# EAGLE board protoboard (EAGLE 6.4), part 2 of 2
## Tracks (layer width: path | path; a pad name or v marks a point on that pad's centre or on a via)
A1
  Top 0.61: PIN1A.1 21.27,84.61 21.93,84.61 21.93,84.6 18.88,84.6
  Bottom 0.254: 21.25,75.25 21.25,75.37 21.21,75.37 21.21,75.27
  Bottom 0.406: 19,75.25 21.25,75.25 | 21.25,75.25 25.47,75.25 | 21.25,75.25 21.25,75.76 21.25,87.92 21.27,87.92
  Bottom 0.61: PIN1A.1 21.25,88.42 21.25,75.76 | 21.25,76.05 21.25,75.37
A2
  Top 0.305: 21.27,83.34 18.73,83.34
  Top 0.61: 21.91,83.34 18.73,83.34 17.46,83.34 17.46,88.42 PIN2A.1
  Bottom 0.254: 18,74.6 18,74.69
  Bottom 0.406: 25.53,74.6 18,74.6 18,74.82 18,88.41
  Bottom 0.61: PIN2A.1 18,88.42 18,74.82 | 18,74.98 18,74.69
A3
  Top 0.61: 21.91,82.07 16.51,82.07 16.51,90.96 PIN3A.1
  Bottom 0.254: 17.02,74.82 17.02,74.79
  Bottom 0.406: 25.47,73.95 17.02,73.95 17.02,74.79 | 18.73,90.98 PIN3A.1
  Bottom 0.61: 18.73,90.98 17.02,90.98 17.02,74.79 | 17.02,74.82 17.02,74.04
A4
  Top 0.61: 21.91,80.8 15.56,80.8 15.56,93.5 PIN4A.1
  Bottom 0.254: 16.05,73.91 16.04,73.91
  Bottom 0.406: 25.47,73.3 16.04,73.3 16.04,73.91 16.04,92.8
  Bottom 0.61: PIN4A.1 16.04,93.5 16.04,73.91 | 16.05,73.91 16.05,73.39
A5
  Top 0.61: 21.91,79.53 14.61,79.53 14.61,91.92 13.65,91.92 PIN5A.1
  Bottom 0.254: 15.07,73.55 15.07,73.52
  Bottom 0.406: 25.47,72.65 15.07,72.65 15.07,73.52 15.07,90.85
  Bottom 0.61: PIN5A.1 13.65,90.84 15.07,90.84 15.07,73.52 | 15.07,73.55 15.07,72.74
A6
  Top 0.61: 21.91,78.26 13.65,78.26 13.65,90.96 PIN6A.1
  Bottom 0.254: 14.1,72 14.1,72.09
  Bottom 0.406: 25.47,72 14.1,72 14.1,72.84
  Bottom 0.61: PIN6A.1 11.11,89.93 14.1,89.93 14.1,72.84 | 14.1,73.1 14.1,72.09
A7
  Top 0.61: 21.91,76.99 12.7,76.99 12.7,88.42 PIN7A.1
  Bottom 0.254: 13.12,71.35 13.12,71.44
  Bottom 0.406: 25.47,71.35 13.12,71.35 13.12,71.8 | PIN7A.1
  Bottom 0.61: PIN7A.1 13.12,88.41 13.12,71.8 | 13.12,71.93 13.12,71.44
A8
  Top 0.61: 21.91,75.72 11.75,75.72 11.75,85.88 PIN8A.1
  Bottom 0.254: 12.15,71.24 12.14,71.24 12.14,71.28
  Bottom 0.406: 25.47,70.7 12.14,70.7 12.14,71.18 | PIN8A.1
  Bottom 0.61: PIN8A.1 12.14,85.88 12.14,71.28 12.14,71.18 | 12.15,71.24 12.15,70.79
A9
  Top 0.61: 21.91,74.45 10.79,74.45 10.79,83.34 PIN9A.1
  Bottom 0.254: 11.17,70.14 11.17,70.17
  Bottom 0.406: 25.47,70.05 11.17,70.05 11.17,70.17 11.17,70.46 | PIN9A.1
  Bottom 0.61: PIN9A.1 11.17,83.34 11.17,70.46 | 11.17,70.66 11.17,70.14
A10
  Top 0.305: 20.64,73.18 19.68,73.18
  Top 0.61: PIN10A.1 9.84,80.8 9.84,73.18 19.68,73.18 21.91,73.18
  Bottom 0.254: 10.2,69.49 10.2,69.52
  Bottom 0.406: 25.47,69.4 10.2,69.4 10.2,69.52 10.2,69.85 10.2,80.81
  Bottom 0.61: PIN10A.1 10.2,80.8 10.2,69.85 | 10.2,69.98 10.2,69.49
A11
  Top 0.61: 21.91,71.91 8.89,71.91 8.89,78.26 PIN11A.1
  Bottom 0.254: 9.22,68.87 9.22,68.94
  Bottom 0.406: 25.47,68.75 9.22,68.75 9.22,68.94 9.22,69.62 9.22,78.27
  Bottom 0.61: PIN11A.1 9.22,78.26 9.22,69.62 | 9.22,69.94 9.22,68.87
A12
  Top 0.61: 21.91,70.64 7.94,70.64 7.94,75.72 PIN12A.1
  Bottom 0.254: 8.25,68.19 8.24,68.19 8.24,68.22
  Bottom 0.406: 25.47,68.1 8.24,68.1 8.24,68.22 8.24,68.87 8.24,75.7
  Bottom 0.61: PIN12A.1 8.24,75.72 8.24,68.87 | 8.25,69 8.25,68.19
A13
  Top 0.305: 6.98,73.18 6.67,73.18
  Top 0.61: 21.91,69.37 6.98,69.37 6.98,73.18 | 6.67,73.18 PIN13A.1 6.07,73.18 6.07,73.17
  Bottom 0.406: 25.47,67.45 7.27,67.45 7.27,67.67 7.27,68.12
  Bottom 0.61: 6.03,73.17 6.1,73.17 | 6.1,73.17 7.27,73.17 7.27,68.12 | 7.27,68.29 7.27,67.67 | 7.27,67.57 7.27,67.67 | 7.27,67.67 | PIN13A.1 6.1,73.18 6.1,73.17
A14
  Top 0.61: 21.91,68.1 6.03,68.1 6.03,70.64 PIN14A.1
  Bottom 0.254: 6.3,66.89 6.29,66.89 6.29,66.95
  Bottom 0.406: 25.47,66.8 6.29,66.8 6.29,66.95 6.29,67.28 6.29,70.63
  Bottom 0.61: PIN14A.1 6.29,70.64 6.29,67.28 | 6.3,67.47 6.3,66.89
A15
  Top 0.61: 21.91,66.83 5.08,66.83 5.08,68.1 PIN15A.1
  Bottom 0.254: 5.32,66.24 5.32,66.27
  Bottom 0.406: 25.47,66.15 5.32,66.15 5.32,66.27 5.32,66.73
  Bottom 0.61: 5.32,66.73 5.32,68.1 PIN15A.1 | 5.32,66.86 5.32,66.24
A16
  Top 0.61: 21.91,65.56 PIN16A.1
  Bottom 0.406: 25.47,65.5 4.9,65.5 4.34,65.5
  Bottom 0.61: PIN16A.1 3.49,65.5 4.9,65.5
A17
  Top 0.61: 21.91,64.29 5.08,64.29 5.08,63.02 PIN17A.1
  Bottom 0.406: 25.47,64.85 5.32,64.85 5.32,64.75
  Bottom 0.61: 5.32,64.75 5.32,63.02 PIN17A.1
A18
  Top 0.61: 21.91,63.02 6.03,63.02 6.03,60.48 PIN18A.1
  Bottom 0.254: 6.3,64.09 6.29,64.09
  Bottom 0.406: 25.47,64.2 6.29,64.2 6.29,64.09 6.29,63.67 6.29,60.62
  Bottom 0.61: PIN18A.1 6.29,60.48 6.29,63.67 | 6.3,63.54 6.3,64.09
A19
  Top 0.61: 21.91,61.75 6.98,61.75 6.98,57.94 PIN19A.1
  Bottom 0.254: 7.27,62.99 7.27,63.02
  Bottom 0.406: 25.47,63.55 7.27,63.55 7.27,63.05 | 7.27,63.02 7.27,58.25
  Bottom 0.61: PIN19A.1 7.27,57.94 7.27,63.02 7.27,63.05 | 7.27,62.99 7.27,63.44
A20
  Top 0.61: 21.91,60.48 7.94,60.48 7.94,55.4 PIN20A.1
  Bottom 0.254: 8.25,62.79 8.24,62.79 8.24,62.76
  Bottom 0.305: 6.03,55.42 PIN20A.1
  Bottom 0.406: 25.47,62.9 8.24,62.9 8.24,62.76 8.24,62.37
  Bottom 0.61: 6.03,55.42 8.24,55.42 8.24,62.37 | 8.25,62.08 8.25,62.79
A21
  Top 0.61: 21.91,59.21 8.89,59.21 8.89,52.86 PIN21A.1
  Bottom 0.254: 9.22,62.25 9.22,62.14
  Bottom 0.406: 25.47,62.25 9.22,62.25 9.22,61.75 9.22,52.82
  Bottom 0.61: PIN21A.1 9.22,52.86 9.22,61.75 | 9.22,61.62 9.22,62.14
A22
  Top 0.61: 21.91,57.94 9.84,57.94 9.84,50.32 PIN22A.1
  Bottom 0.254: 10.2,61.49 10.29,61.49 10.29,61.6
  Bottom 0.406: 25.47,61.6 10.29,61.6 10.2,61.6 10.2,61.1 10.2,50.45
  Bottom 0.61: PIN22A.1 10.2,50.32 10.2,61.1 | 10.2,60.88 10.2,61.49
A23
  Top 0.61: 21.91,56.67 10.79,56.67 10.79,47.78 PIN23A.1
  Bottom 0.254: 11.17,60.45 11.17,60.49
  Bottom 0.406: 25.47,60.95 11.17,60.95 11.17,60.49 11.17,60.42 11.17,47.95
  Bottom 0.61: PIN23A.1 11.17,47.78 11.17,60.42 | 11.17,60.45 11.17,60.84
A24
  Top 0.61: 21.91,55.4 11.75,55.4 11.75,45.24 9.21,45.24 PIN24A.1
  Bottom 0.254: 12.14,59.8 12.15,59.8 12.15,59.77
  Bottom 0.406: 25.47,60.3 12.14,60.3 12.14,59.8
  Bottom 0.61: PIN24A.1 12.14,45.24 12.14,59.8 | 12.15,59.71 12.15,59.77 12.15,60.19
A25
  Top 0.61: 21.91,54.13 12.7,54.13 12.7,42.7 PIN25A.1
  Bottom 0.254: 13.12,59.06 13.12,59.02
  Bottom 0.406: 25.47,59.65 13.12,59.65 13.12,59.06 13.12,42.75
  Bottom 0.61: PIN25A.1 13.12,42.7 13.12,59.06 | 13.12,59.02 13.12,59.54
A26
  Top 0.61: 21.91,52.86 13.65,52.86 13.65,40.16 PIN26A.1
  Bottom 0.254: 14.1,58.5 14.1,58.57
  Bottom 0.406: 25.47,59 14.1,59 14.1,58.5
  Bottom 0.61: PIN26A.1 11.11,41.45 14.1,41.45 14.1,58.5 | 14.1,58.57 14.1,58.89
A27
  Top 0.61: 21.84,51.59 14.61,51.59 14.61,39.21 13.65,39.21 PIN27A.1
  Bottom 0.254: 15.07,57.92 15.07,57.98
  Bottom 0.406: 25.47,58.35 15.07,58.35 15.07,57.98 15.07,40.47
  Bottom 0.61: PIN27A.1 13.65,40.47 15.07,40.47 15.07,57.98 | 15.07,57.92 15.07,58.24
A28
  Top 0.61: 21.84,50.32 15.56,50.32 15.56,37.62 PIN28A.1
  Bottom 0.254: 16.05,57.11 16.04,57.11 16.04,57.17
  Bottom 0.406: 25.47,57.7 16.04,57.7 16.04,57.17 16.04,38.52
  Bottom 0.61: PIN28A.1 16.04,37.62 16.04,57.17 | 16.05,57.11 16.05,57.59
A29
  Top 0.61: 21.84,49.05 16.51,49.05 16.51,40.16 PIN29A.1
  Bottom 0.254: 17.02,56.94
  Bottom 0.305: 17.05,57.04 17.02,57.04 17.02,56.99
  Bottom 0.406: 17.02,57.05 17.02,56.99 17.02,56.94 17.02,56.49 17.02,40.15 | 17.05,57.04 25.44,57.04
  Bottom 0.61: PIN29A.1 17.02,40.16 17.02,56.49 | 17.02,56.42 17.02,56.94
A30
  Top 0.61: 21.84,47.78 17.46,47.78 17.46,42.7 PIN30A.1
  Bottom 0.254: 18,55.87
  Bottom 0.305: 18,56.4 18.03,56.4 18.03,56.39
  Bottom 0.406: 18,56.4 18,55.87 18,42.75 | 18.03,56.39 25.44,56.39
  Bottom 0.61: PIN30A.1 18,42.7 18,55.87 | 18,55.87 18,56.29
A31
  Top 0.61: 18.67,46.51 21.27,46.51 | 21.27,46.51 21.91,46.51 | PIN31A.1 21.27,46.51
  Bottom 0.254: 21.21,55.74 21.25,55.74 21.25,55.58
  Bottom 0.305: 21.25,55.75 21.27,55.75 21.27,55.74
  Bottom 0.406: 18.97,55.75 21.25,55.75 21.25,55.25 21.25,43.72 | 21.21,55.74 21.27,55.74 25.44,55.74
  Bottom 0.61: PIN31A.1 21.25,42.7 21.25,55.25 | 21.25,54.99 21.25,55.58
B1
  Top 0.61: 33.97,84.61 31.43,84.61 | 31.43,84.61 23.18,84.61 | 31.43,84.61 PIN1B.1
  Bottom 0.254: 31.64,76.15 31.65,76.15
  Bottom 0.406: 27.42,75.25 31.64,75.25 | 31.64,75.25 34.19,75.25 | 31.64,87.6 31.64,76.15 31.64,75.25
  Bottom 0.61: PIN1B.1 31.64,88.42 31.64,76.15 | 31.65,76.15 31.65,75.44
B2
  Top 0.61: 23.18,83.34 35.24,83.34 35.24,88.42 PIN2B.1
  Bottom 0.254: 34.9,76.15 34.9,76.12
  Bottom 0.406: 27.42,74.6 34.9,74.6 34.9,76.15 34.9,88.25
  Bottom 0.61: PIN2B.1 34.9,88.42 34.9,76.15 | 34.9,76.51 34.9,76.12 34.9,75.7
B3
  Top 0.61: PIN3B.1 36.2,90.96 36.2,82.07 23.18,82.07
  Bottom 0.254: 35.87,74.75
  Bottom 0.406: 27.42,73.95 35.87,73.95 35.87,74.75 35.87,90.85
  Bottom 0.61: PIN3B.1 35.87,90.96 35.87,74.75 | 35.87,74.82 35.87,74.75 35.87,74.04
B4
  Top 0.61: 23.18,80.8 37.15,80.8 37.15,93.5 PIN4B.1
  Bottom 0.254: 36.85,74.07 36.85,74.01
  Bottom 0.406: 27.42,73.3 36.85,73.3 36.85,74.07 36.85,92.8
  Bottom 0.61: PIN4B.1 36.85,93.5 36.85,74.07 | 36.85,74.1 36.85,74.01 36.85,73.39
B5
  Top 0.61: 23.18,79.53 38.1,79.53 38.1,91.92 39.05,91.92 PIN5B.1
  Bottom 0.406: 27.42,72.65 37.82,72.65 37.82,73.62 37.82,90.85
  Bottom 0.61: PIN5B.1 39.05,91.49 37.82,91.49 37.82,73.62 | 37.82,73.62 | 37.82,73.62 37.82,72.74
B6
  Top 0.61: PIN6B.1 39.05,90.96 39.05,78.26 23.18,78.26
  Bottom 0.254: 38.8,72.41 38.8,72.45
  Bottom 0.406: 27.42,72 38.8,72 38.8,72.41 38.8,89.55
  Bottom 0.61: PIN6B.1 41.59,89.54 38.8,89.54 38.8,72.41 | 38.8,72.45 38.8,72.09
B7
  Top 0.61: PIN7B.1 40.01,88.42 40.01,76.99 23.18,76.99
  Bottom 0.254: 39.77,71.35 39.77,71.44
  Bottom 0.406: 27.42,71.35 39.77,71.35 39.77,72.28 39.77,88.25
  Bottom 0.61: PIN7B.1 39.77,88.42 39.77,72.28 | 39.77,73.36 39.77,71.44
B8
  Top 0.61: 23.18,75.72 40.96,75.72 40.96,85.88 PIN8B.1
  Bottom 0.406: 27.42,70.7 40.75,70.7 40.75,70.79 40.75,85.97
  Bottom 0.61: PIN8B.1 40.75,85.88 40.75,70.79
B9
  Top 0.61: 23.18,74.45 41.91,74.45 41.91,83.34 PIN9B.1
  Bottom 0.254: 41.72,70.05 41.72,70.14
  Bottom 0.406: 27.42,70.05 41.72,70.05 41.72,70.82 | PIN9B.1 44.13,83.37
  Bottom 0.61: 44.13,83.37 41.72,83.37 41.72,70.82 | 41.72,70.95 41.72,70.14
B10
  Top 0.61: 23.18,73.18 42.86,73.18 42.86,80.8 PIN10B.1
  Bottom 0.254: 42.7,69.49 42.7,69.46
  Bottom 0.406: 27.42,69.4 42.7,69.4 42.7,69.46 42.7,69.85 | 44.13,80.77 PIN10B.1
  Bottom 0.61: 44.13,80.77 42.7,80.77 42.7,69.85 | 42.7,69.98 42.7,69.49
B11
  Top 0.61: 23.18,71.91 43.82,71.91 43.82,78.26 PIN11B.1
  Bottom 0.305: 46.67,78.17 PIN11B.1
  Bottom 0.406: 27.42,68.75 43.67,68.75 43.67,78.17
  Bottom 0.61: 43.67,78.17 45.95,78.17 46.67,78.17
B12
  Top 0.61: 23.18,70.64 44.77,70.64 44.77,75.72 PIN12B.1
  Bottom 0.254: 44.65,68.19
  Bottom 0.406: 27.42,68.1 44.65,68.1 44.65,68.19 44.65,68.58 44.65,75.57
  Bottom 0.61: PIN12B.1 44.65,75.72 44.65,68.58 | 44.65,68.81 44.65,68.19
B13
  Top 0.61: 23.18,69.37 45.72,69.37 45.72,73.18 PIN13B.1
  Bottom 0.254: 45.62,68.09
  Bottom 0.406: 27.42,67.45 45.62,67.45 45.62,68.03 | 45.62,68.09 45.62,72.65
  Bottom 0.61: PIN13B.1 45.62,73.18 45.62,68.09 45.62,68.03 | 45.62,68.09 45.62,67.54
B14
  Top 0.61: 23.18,68.1 46.67,68.1 46.67,70.64 PIN14B.1
  Bottom 0.254: 46.6,66.89
  Bottom 0.406: 27.42,66.8 46.6,66.8 46.6,66.89 46.6,67.31 46.6,70.7
  Bottom 0.61: PIN14B.1 46.6,70.64 46.6,67.31 | 46.6,67.54 46.6,66.89
B15
  Top 0.61: 23.18,66.83 47.62,66.83 47.62,68.1 PIN15B.1
  Bottom 0.254: 47.57,66.73 47.57,66.69
  Bottom 0.406: 27.42,66.15 47.57,66.15 47.57,66.63 | PIN15B.1
  Bottom 0.61: PIN15B.1 47.57,68.1 47.57,66.69 47.57,66.63 | 47.57,66.73 47.57,66.24
B16
  Top 0.61: 23.18,65.56 PIN16B.1
  Bottom 0.406: 27.42,65.5 48,65.5 48.55,65.5 | 49.21,65.5 PIN16B.1
  Bottom 0.61: 49.21,65.5 48,65.5
B17
  Top 0.61: 23.18,64.29 47.62,64.29 47.62,63.02 PIN17B.1
  Bottom 0.254: 47.57,64.29 47.57,64.26
  Bottom 0.406: 27.42,64.85 47.57,64.85 47.57,64.65 | 47.57,64.26 47.57,63.09
  Bottom 0.61: PIN17B.1 47.57,63.02 47.57,64.26 47.57,64.65 | 47.57,64.29 47.57,64.74
B18
  Top 0.61: 23.18,63.02 46.67,63.02 46.67,60.48 PIN18B.1
  Bottom 0.254: 46.6,64.2 46.6,64.09
  Bottom 0.406: 27.42,64.2 46.6,64.2 46.6,63.31 46.6,60.82
  Bottom 0.61: PIN18B.1 46.6,60.48 46.6,63.31 | 46.6,62.89 46.6,64.09
B19
  Top 0.61: 23.18,61.75 45.72,61.75 45.72,57.94 PIN19B.1
  Bottom 0.254: 45.62,62.96 45.62,62.99
  Bottom 0.406: 27.42,63.55 45.62,63.55 45.62,62.96 45.62,58.35
  Bottom 0.61: PIN19B.1 45.62,57.94 45.62,62.96 | 45.62,62.89 45.62,62.99 45.62,63.44
B20
  Top 0.61: 23.18,60.48 44.77,60.48 44.77,55.4 PIN20B.1
  Bottom 0.254: 44.65,62.9 44.65,62.79
  Bottom 0.406: 27.42,62.9 44.65,62.9 44.65,62.44 44.65,55.42
  Bottom 0.61: PIN20B.1 44.65,55.4 44.65,62.44 | 44.65,62.24 44.65,62.79
B21
  Top 0.61: PIN21B.1 43.82,52.86 43.82,59.21 23.18,59.21
  Bottom 0.254: 43.67,62.25 43.67,62.14
  Bottom 0.406: 27.42,62.25 43.67,62.25 43.67,61.75 43.67,53.31 | 46.67,52.82 PIN21B.1
  Bottom 0.61: 46.67,52.82 43.67,52.82 43.67,61.75 | 43.67,61.53 43.67,62.14
B22
  Top 0.61: 23.18,57.94 42.86,57.94 42.86,50.32 PIN22B.1
  Bottom 0.254: 42.7,61.6 42.7,61.49
  Bottom 0.406: 27.42,61.6 42.7,61.6 42.7,60.75 42.7,50.55
  Bottom 0.61: PIN22B.1 42.7,50.32 42.7,60.75 | 42.7,60.26 42.7,61.49
B23
  Top 0.61: PIN23B.1 41.91,47.78 41.91,56.67 23.18,56.67
  Bottom 0.254: 41.72,60.84 41.72,60.88
  Bottom 0.406: 27.42,60.95 41.72,60.95 41.72,60.88 41.72,60.52 41.72,47.95
  Bottom 0.61: PIN23B.1 41.72,47.78 41.72,60.52 | 41.72,60.19 41.72,60.84
B24
  Top 0.61: 23.18,55.4 40.96,55.4 40.96,45.24 PIN24B.1
  Bottom 0.254: 40.75,60.3 40.75,60.19
  Bottom 0.406: 27.42,60.3 40.75,60.3 40.75,59.8 40.75,45.35
  Bottom 0.61: PIN24B.1 40.75,45.24 40.75,59.8 | 40.75,59.48 40.75,60.19
B25
  Top 0.61: PIN25B.1 40.01,42.7 40.01,54.13 23.18,54.13
  Bottom 0.254: 39.77,59.65 39.77,59.54
  Bottom 0.406: 27.42,59.65 39.77,59.65 39.77,59.15 39.77,43.07
  Bottom 0.61: PIN25B.1 39.77,42.7 39.77,59.15 | 39.77,58.86 39.77,59.54
B26
  Top 0.61: 23.18,52.86 39.05,52.86 39.05,40.16 PIN26B.1
  Bottom 0.254: 38.8,59 38.8,58.89
  Bottom 0.406: 27.42,59 38.8,59 38.8,58.54 38.8,41.45
  Bottom 0.61: PIN26B.1 41.59,41.44 38.8,41.44 38.8,58.54 | 38.8,58.34 38.8,58.89
B27
  Top 0.61: 23.18,51.59 38.1,51.59 38.1,38.89 39.05,38.89 PIN27B.1
  Bottom 0.254: 37.82,58.35 37.82,58.24
  Bottom 0.406: 27.42,58.35 37.82,58.35 37.82,57.85 37.82,40.15
  Bottom 0.61: PIN27B.1 39.05,40.14 37.82,40.14 37.82,57.85 | 37.82,57.72 37.82,58.24
B28
  Top 0.61: 23.18,50.32 37.15,50.32 37.15,37.62 PIN28B.1
  Bottom 0.254: 36.85,57.59 36.85,57.63
  Bottom 0.406: 27.42,57.7 36.85,57.7 36.85,57.63 36.85,57.37 36.85,38.2
  Bottom 0.61: PIN28B.1 36.85,37.62 36.85,57.37 | 36.85,57.24 36.85,57.59
B29
  Top 0.61: 23.18,49.05 36.2,49.05 36.2,40.16 PIN29B.1 34.02,40.16 34.02,40.15 | 34.02,40.15 33.97,40.15 | 35.03,40.15 34.54,40.15 34.02,40.15
  Bottom 0.254: 33.97,40.15 PIN29B.1
  Bottom 0.406: 34.57,40.15 35.87,40.15 35.87,57.05 35.88,57.05 35.88,56.36 35.91,56.36 35.91,56.42 | 27.45,57.04 35.91,57.04 35.91,56.94
  Bottom 0.61: 33.97,40.15 35.91,40.15 35.91,56.42 35.91,56.94
B30
  Top 0.61: 23.18,47.78 35.24,47.78 35.24,42.7 PIN30B.1
  Bottom 0.254: 34.9,56.39 34.9,56.4
  Bottom 0.406: 34.9,56.39 27.45,56.39 | 34.9,56.4 34.9,55.29 34.9,43.07
  Bottom 0.61: PIN30B.1 34.9,42.7 34.9,55.29
B31
  Top 0.61: PIN31B.1 31.43,46.51 | 31.43,46.51 33.97,46.51 | 23.18,46.51 31.43,46.51
  Bottom 0.254: 31.65,55.58 31.65,55.74 31.65,55.75
  Bottom 0.406: 34.12,55.75 31.65,55.75 31.64,55.75 31.64,55.42 31.64,43.4 | 31.75,55.74 31.65,55.74 27.45,55.74
  Bottom 0.61: PIN31B.1 31.64,42.7 31.64,55.42 | 31.65,54.8 31.65,55.58
BOK1  (via drill 0.7)
  Top 2.184: 11.11,93.82 v11.11,97.31
  Bottom 0.406: PIN-BOK1.1 11.17,93.5 11.17,93.28 11.11,93.28 11.11,93.82
  Bottom 2.184: v11.11,97.31 11.11,93.82
BOK2  (via drill 0.7)
  Top 2.184: 18.73,93.82 v18.73,97.31
  Bottom 0.406: PIN-BOK2.1 18.73,93.82
  Bottom 2.184: v18.73,97.31 18.73,93.82
BOK3  (via drill 0.7)
  Top 2.184: 21.27,93.82 v21.27,97.31
  Bottom 0.406: PIN-BOK3.1 21.27,93.82
  Bottom 2.184: v21.27,97.31 21.27,93.82
BOK4  (via drill 0.7)
  Top 2.184: 23.81,93.82 v23.81,97.31
  Bottom 0.406: PIN-BOK4.1 23.81,93.82
  Bottom 2.184: v23.81,97.31 23.81,93.82
BOK5  (via drill 0.7)
  Top 2.184: 26.35,93.82 v26.35,97.31
  Bottom 0.406: PIN-BOK5.1 26.35,93.82
  Bottom 2.184: v26.35,97.31 26.35,93.82
BOK6  (via drill 0.7)
  Top 2.184: 28.89,93.82 v28.89,97.31
  Bottom 0.61: 28.89,96.04 PIN-BOK6.1 v28.89,97.31
  Bottom 2.184: v28.89,97.31 28.89,96.04 28.89,93.82
BOK7  (via drill 0.7)
  Top 2.184: 31.43,93.82 v31.43,97.31
  Bottom 2.184: v31.43,97.31 PIN-BOK7.1
BOK8  (via drill 0.7)
  Top 2.184: PIN-BOK8.1 v33.97,97.31
  Bottom 2.184: v33.97,97.31 33.97,93.82
BOK9  (via drill 0.7)
  Top 2.184: PIN-BOK9.1 v41.59,97.31
  Bottom 2.184: v41.59,97.31 41.59,93.82
BOK10  (via drill 0.7)
  Top 2.184: PIN-BOK10.1 v44.13,97.31
  Bottom 2.184: v44.13,97.31 44.13,93.82
BOK11  (via drill 0.7)
  Top 2.184: PIN-BOK11.1 v46.67,97.31
  Bottom 2.184: v46.67,97.31 46.67,93.82
BOK12  (via drill 0.7)
  Top 2.184: PIN-BOK12.1 v49.21,97.31
  Bottom 2.184: v49.21,97.31 49.21,93.82
C1
  Top 0.61: IC2.4 18.73,30.95 18.73,32.44 16.19,32.44 PIN1C.1
  Bottom 0.305: 22.32,32.44 22.32,30.84 22.32,23.34 22.54,23.34 | 22.32,23.34 22.54,23.34 | 22.54,23.34 31.96,23.34
  Bottom 0.61: PIN1C.1 22.32,32.54 22.32,30.84
C2
  Top 0.61: IC2.5 PIN2C.1
  Bottom 0.305: 21.91,22.83 21.59,22.83 | 21.59,22.83 21.53,22.83 21.53,28.34 | 31.96,22.84 21.59,22.84 21.59,22.83
  Bottom 0.61: PIN2C.1 21.53,30 21.53,28.34
C3
  Top 0.61: IC2.6 18.73,29.05 18.73,27.56 16.19,27.56 PIN3C.1
  Bottom 0.254: PIN3C.1
  Bottom 0.305: 20.82,25.84 20.82,22.34 31.96,22.34
  Bottom 0.61: PIN3C.1 20.82,27.47 20.82,25.84
C4
  Top 0.813: PIN4C.1 29.53,24.92 U6.P_POUZDRO
  Bottom 0.254: PIN4C.1 16.96,24.92 16.96,24.94
  Bottom 0.305: 20.07,23.84 20.07,21.84 20.32,21.84 | 20.07,21.84 20.32,21.84 | 20.32,21.84 31.96,21.84
  Bottom 0.61: 16.19,24.94 16.96,24.94 20.07,24.94 20.07,23.84
C5
  Top 0.813: PIN5C.1 23.33,22.38 U6.P_A
  Bottom 0.305: 19.32,22.38 19.32,21.84 19.32,21.34 31.96,21.34
  Bottom 0.61: PIN5C.1 19.32,22.38 19.32,21.84
C6
  Top 0.813: U6.P-B PIN6C.1
  Bottom 0.254: PIN6C.1 16.46,19.84 16.46,19.81
  Bottom 0.305: 19.32,20.34 19.32,20.84 31.96,20.84
  Bottom 0.61: 16.19,19.81 16.46,19.81 19.32,19.81 19.32,20.34
C7
  Top 0.813: PIN7C.1 23.33,17.3 U6.P-C
  Bottom 0.254: PIN7C.1 16.46,17.3 16.46,17.31
  Bottom 0.305: 20.07,20.34 20.07,18.84 | 20.07,20.35 20.07,20.34 | 20.07,20.34 31.96,20.34
  Bottom 0.61: 16.19,17.31 16.46,17.31 20.07,17.31 20.07,18.84
C8
  Top 0.61: U1.1 18.41,13.8 18.41,14.69 16.19,14.69 PIN8C.1
  Bottom 0.254: PIN8C.1
  Bottom 0.305: 20.82,15.84 20.82,19.84 31.96,19.84
  Bottom 0.61: PIN8C.1 20.82,14.75 20.82,15.84
C9
  Top 0.61: U1.2 PIN9C.1
  Bottom 0.254: 16.19,12.19 PIN9C.1
  Bottom 0.305: 21.57,13.84 21.57,19.34 31.96,19.34
  Bottom 0.61: 16.19,12.19 21.57,12.19 21.57,13.84
C10
  Top 0.61: U1.3 18.41,10.52 18.41,9.56 16.16,9.56 PIN10C.1
  Bottom 0.305: 22.32,9.66 22.32,11.34 22.32,18.83 31.96,18.83 31.96,18.84
  Bottom 0.61: PIN10C.1 22.32,9.65 22.32,11.34
D1
  Top 0.406: IC1.3 46.04,30.65 46.04,31.59 | 49.21,32.6 PIN1D.1
  Top 0.61: 46.04,31.59 46.04,32.6 49.21,32.6
  Bottom 0.254: PIN1D.1
  Bottom 0.305: 43.82,31.34 43.82,23.34 32.78,23.34
  Bottom 0.61: PIN1D.1 43.82,32.53 43.82,31.34
D2
  Top 0.406: IC1.2 46.67,30
  Top 0.61: PIN2D.1 46.67,30
  Bottom 0.254: PIN2D.1
  Bottom 0.305: 44.57,29.34 44.57,22.84 32.78,22.84
  Bottom 0.61: PIN2D.1 44.57,30 44.57,29.34
D3
  Top 0.406: IC1.1 46.04,29.35 46.04,28.26
  Top 0.61: 46.04,28.26 46.04,27.46 PIN3D.1
  Bottom 0.305: 45.28,26.84 45.28,22.34 32.78,22.34
  Bottom 0.61: PIN3D.1 45.28,27.46 45.28,26.84
D4
  Top 0.813: U7.P_POUZDRO 34.72,24.92 PIN4D.1
  Bottom 0.305: 46.07,24.91 46.07,23.84 46.07,21.84 32.78,21.84
  Bottom 0.61: PIN4D.1 46.07,24.92 46.07,23.84
D5
  Top 0.813: U7.P-A 42.02,22.38 PIN5D.1
  Bottom 0.305: 46.82,22.38 46.82,21.84 46.82,21.34 32.78,21.34
  Bottom 0.61: PIN5D.1 46.82,22.38 46.82,21.84
D6
  Top 0.813: U7.P-B PIN6D.1
  Bottom 0.254: PIN6D.1 48.97,19.84
  Bottom 0.305: 46.82,20.34 46.82,20.81 46.67,20.81 46.67,20.84 | 46.82,20.84 46.67,20.84 | 46.67,20.84 32.78,20.84
  Bottom 0.61: PIN6D.1 48.97,19.84 46.82,19.84 46.82,20.34
D7
  Top 0.813: U7.P-C 42.02,17.3 PIN7D.1
  Bottom 0.305: 46.07,17.31 46.07,18.84 46.07,20.34 32.78,20.34
  Bottom 0.61: PIN7D.1 46.07,17.3 46.07,18.84
D8
  Top 0.61: U2.6 46.04,13.92 46.04,14.81 49.21,14.81 PIN8D.1
  Bottom 0.254: PIN8D.1 48.97,14.76 48.97,14.75
  Bottom 0.305: 45.32,15.84 45.32,19.81 45.09,19.81 45.09,19.84 | 32.78,19.84 45.09,19.84 | 45.09,19.84 45.32,19.84
  Bottom 0.61: PIN8D.1 48.97,14.75 45.32,14.75 45.32,15.84
D9
  Top 0.61: U2.5 PIN9D.1
  Bottom 0.254: PIN9D.1 48.97,12.22
  Bottom 0.305: 44.57,13.34 44.57,19.31 44.45,19.31 44.45,19.34 | 44.57,19.34 44.45,19.34 | 44.45,19.34 32.78,19.34
  Bottom 0.61: PIN9D.1 48.97,12.22 44.57,12.22 44.57,13.34
D10
  Top 0.61: U2.4 46.36,10.52 46.36,9.69 PIN10D.1
  Bottom 0.305: 43.82,9.69 43.82,10.84 43.82,18.84 32.78,18.84
  Bottom 0.61: PIN10D.1 43.82,9.68 43.82,10.84
IO/A
  Bottom 1.27: ARK-A.1 K1.1
IO/B
  Bottom 1.27: ARK-B.1 K1.2
IO/C
  Top 0.813: J-LED1A.1 84.77,96.52 K1.3
  Bottom 1.27: ARK-C.1 K1.3
IO/D
  Top 0.813: J-LED2A.1 66.99,93.98 66.99,95.41 79.69,95.41 K2.1
  Bottom 1.27: ARK-D.1 K2.1
IO/E
  Top 0.813: ARK-E.1 74.61,89.38 66.99,89.38 66.99,91.44 J-LED3A.1
  Bottom 1.27: ARK-E.1 K2.2
IO/F
  Top 0.813: ARK-F.1 65.09,86.04 J-LED4A.1
  Bottom 1.27: ARK-F.1 K2.3
J-2MM-A1  (via drill 0.9 pad 1.68)
  other vias: 8.2,38.32
J-2MM-A2  (via drill 0.9 pad 1.68)
  other vias: 8.2,36.32
J-2MM-A3  (via drill 0.9 pad 1.68)
  other vias: 8.2,34.32
J-2MM-A4  (via drill 0.9 pad 1.68)
  other vias: 8.2,32.33
J-2MM-B1  (via drill 0.9 pad 1.68)
  other vias: 3.2,38.32
J-2MM-B2  (via drill 0.9 pad 1.68)
  other vias: 3.2,36.32
J-2MM-B3  (via drill 0.9 pad 1.68)
  other vias: 3.19,34.33
J-2MM-B4  (via drill 0.9 pad 1.68)
  other vias: 3.2,32.32
LED1A
  Top 1.27: LED1.A J-LED1B.1
  Top 1.422: 59.37,96.52 LED1.A
LED2A
  Top 1.27: LED2.A J-LED2B.1
  Top 1.422: LED2.A 59.37,93.98
LED3A
  Top 1.27: LED3.A J-LED3B.1
  Top 1.422: LED3.A 59.37,91.44
LED4A
  Top 1.27: LED4.A J-LED4B.1
  Top 1.422: LED4.A 59.37,88.9
LEDK1
  Top 1.27: RLED1.2 LED1.C
LEDK2
  Top 1.27: RLED2.2 LED2.C
LEDK3
  Top 1.27: RLED3.2 LED3.C
LEDK4
  Top 1.27: RLED4.2 LED4.C
LEDNAP-K
  Top 1.27: LED-NAP.C RLED-NAP.2
POT1
  Bottom 0.813: PINPOT1B.1 PINPOT1A.1
POT2
  Bottom 0.813: PINPOT2B.1 PINPOT2A.1
SOT1
  Top 0.61: IC2.3 24.13,30.95 24.13,32.54 PIN-SOT1.1
SOT2
  Top 0.406: 23.81,30 24.66,30 25.4,30
  Top 0.61: IC2.2 24.66,30 PIN-SOT2.1
SOT3
  Top 0.406: 24.45,27.46 25.4,27.46
  Top 0.61: IC2.1 23.81,29.05 23.81,27.46 24.45,27.46 PIN-SOT3.1
SOT4
  Top 0.61: U1.6 26.67,13.92 26.67,14.76 PIN-SOT4.1
SOT5
  Top 0.61: U1.5 PIN-SOT5.1
SOT6
  Top 0.61: U1.4 26.67,10.52 26.67,9.68 PIN-SOT6.1
SOT7
  Top 0.406: IC1.4 41.59,30.65 41.59,31.75
  Top 0.61: PIN-SOT7.1 41.59,32.54 41.59,31.75
SOT8
  Top 0.406: 40.8,30 40.8,29.99 | 39.05,29.99 PIN-SOT8.1 | IC1.5 40.32,29.99
  Top 0.61: 40.8,29.99 40.32,29.99 39.05,29.99
SOT9
  Top 0.406: IC1.6 41.59,29.35 41.59,28.26
  Top 0.61: PIN-SOT9.1 41.59,27.46 41.59,28.26
SOT10
  Top 0.61: U2.1 38.42,13.8 38.42,14.76 PIN-SOT10.1
SOT11
  Top 0.61: U2.2 PIN-SOT11.1
SOT12
  Top 0.61: U2.3 38.42,10.52 38.42,9.68 PIN-SOT12.1
TINY-B0
  Bottom 1.27: JP24.1 J-B4.1
TINY-B1
  Bottom 1.27: JP21.1 J-B5.1
TINY-B2
  Bottom 1.27: JP20.1 J-B6.1
TINY-B3
  Bottom 1.27: JP9.1 J-B9.1
TINY-B4
  Bottom 1.27: JP25.1 J-B8.1
TINY-B5
  Bottom 1.27: JP19.1 J-B7.1
TINY/GND  (via drill 0.7)
  Top 0.406: JP117.1 94.93,4.6
  Top 0.813: 69.69,2.38 84.14,2.38 84.14,2.54 ATTINY.4 | 69.69,2.38 58.9,2.38 | 58.9,2.38 57.31,2.38 | 67.15,2.4 67.15,2.86 | 67.15,2.86 58.9,2.86 58.9,2.38 | 67.15,2.86 67.63,2.86 | 69.69,2.38 69.69,20.8 | 69.69,20.8 72.55,20.8 72.55,20.16 69.53,20.16 | 69.69,20.8 69.37,20.8 | 69.53,20.16 69.06,20.16 69.06,20.8 69.37,20.8 | 68.9,20.8 68.74,20.8 68.74,19.37 69.53,19.37 69.53,20.16 | 69.37,20.8 69.37,20.64 69.53,20.64 69.53,20.16 | 57.31,2.38 57.31,35.24 PINGND-10.1 | ATTINY.4 84.14,6.19 | ATTINY.4 84.14,8.57 | RLED-NAP.1 86.68,2.54 | 57.31,2.38 36.51,2.38 | 36.51,2.38 18.73,2.38 PINGND-6.1 PINGND-5.1 | PINGND-8.1 PINGND-7.1 36.51,2.38 | v51.88,80.3 51.75,80.3 JP198.1 51.75,86.52 53.02,86.52 RLED4.1
  Top 1.27: 92.39,4.6 92.39,2.54 86.68,2.54 84.14,2.54 | 92.39,4.6 TINY-ISP.6 | 94.93,4.6 92.39,4.6 | RLED1.1 RLED2.1 RLED3.1 RLED4.1 | PINGND-11.1 PINGND-12.1 PINGND-13.1 PINGND-14.1 PINGND-10.1 PINGND-9.1
  Bottom 0.305: PINGND-4.1 36.51,25.88
  Bottom 0.813: 36.51,27.15 36.51,25.88 36.51,25.24 41.91,25.24 41.91,34.74 | 41.91,34.74 41.91,34.77 12.06,34.77 12.06,29.91 5.71,29.91 5.71,39.21 | 53.97,35.35 53.97,34.74 41.91,34.74 | 53.97,35.35 54.29,35.35 | 53.97,35.35 53.97,36.34
  Bottom 1.016: PINGND-1.1 PINGND-2.1 PINGND-3.1 PINGND-4.1
  Bottom 1.27: TINY-ISP.6 94.93,7.3 C8.2 | PINGND-11.1 PINGND-14.1 54.29,35.35
  Bottom 1.422: PINGND-10.1 51.88,35.24 v51.88,80.3
TINY/MISO/PB1
  Top 0.813: ATTINY.6 82.87,14.92 84.77,16.83 JP28.1
  Bottom 1.27: TINY-ISP.1 84.77,12.38 JP28.1
TINY/MOSI/PB0
  Top 0.406: 87.31,17.62 JP27.1
  Top 0.813: 94.77,9.84 94.77,15.56 87.31,15.56 | 87.31,15.56 JP27.1 | 87.31,15.56 85.73,15.56 85.73,12.84 ATTINY.5 84.14,14.45
  Top 1.016: TINY-ISP.4 94.77,9.84
TINY/PB3
  Top 0.813: ATTINY.2 81.6,4.29 | 81.6,4.29 81.6,3.81 78.11,3.81 78.11,8.89 74.61,12.38 74.61,16.03 | 81.6,4.29 JP96.1
  Top 1.27: JP31.1 74.61,16.03
  Bottom 1.27: P-U/PB3.1 71.6,17.46 JP31.1
TINY/PB4
  Top 0.813: 77.15,16.03 77.15,12.22 79.53,9.84 82.87,9.84 ATTINY.3 82.87,6.19
  Top 1.27: JP32.1 77.15,16.03
  Bottom 1.27: P-U/PB4.1 72.55,14.61 77.15,14.61 JP32.1
TINY/RES/PB5  (via drill 0.7)
  Top 0.813: ATTINY.1 80.33,5.4 v79.69,5.4
  Bottom 0.813: 79.69,15.24 79.69,7.3
  Bottom 1.27: v79.69,5.4 79.69,7.3 TINY-ISP.5 | JP30.1 79.69,15.24
TINY/SCK/PB2
  Top 0.813: ATTINY.7 81.6,16.83 JP29.1
  Bottom 1.27: JP29.1 82.23,9.84 TINY-ISP.3
TINY/SOIC1
  Top 0.813: EMPTY1.1 59.37,9.23 J-SOIC-1.1
  Bottom 0.406: EMPTY2.8 60.69,6.99 59.37,6.99 59.37,6.35
  Bottom 0.813: 59.37,6.35 59.37,10.16 | 59.37,10.16 59.69,10.16 | 59.37,10.16 59.06,10.16
  Bottom 1.27: J-SOIC-1.1 59.37,6.35
TINY/SOIC2
  Top 0.813: EMPTY1.2 63.18,7.46 61.91,6.19 J-SOIC-2.1
  Bottom 0.406: EMPTY2.7 63.44,6.83 61.91,6.83 61.91,6.35 J-SOIC-2.1
  Bottom 1.27: 61.91,4.6 61.91,6.35
TINY/SOIC3
  Top 0.813: EMPTY1.3 J-SOIC-3.1
  Bottom 0.406: EMPTY2.6 64.07,4.76
  Bottom 0.61: J-SOIC-3.1 64.07,4.76
  Bottom 1.27: J-SOIC-3.1 64.45,6.35
TINY/SOIC4
  Top 0.813: EMPTY1.4 66.99,9.23 J-SOIC-4.1
  Bottom 0.406: 66.99,6.35 66.99,6.83 64.72,9.1 EMPTY2.5
  Bottom 1.27: 66.99,6.35 J-SOIC-4.1
TINY/SOIC5
  Top 0.813: EMPTY1.5 66.99,13.95 SOIC-5.1
  Bottom 0.406: EMPTY2.4 64.71,16.76 66.99,19.05
  Bottom 1.27: 66.99,18.57 66.99,19.05 SOIC-5.1
TINY/SOIC6
  Top 0.813: J-SOIC-6.1 EMPTY1.6
  Bottom 0.406: EMPTY2.3 64.07,18.42 64.29,18.42 64.45,18.57
  Bottom 1.27: J-SOIC-6.1 64.45,18.57
TINY/SOIC7
  Top 0.813: J-SOIC-7.1 61.91,17.15 63.18,15.88 EMPTY1.7
  Bottom 0.406: EMPTY2.2 63.44,16.73 61.91,18.26 61.91,18.57
  Bottom 1.27: J-SOIC-7.1 61.91,18.57
TINY/SOIC8
  Top 0.813: EMPTY1.8 59.37,13.95 | 59.37,13.95 J-SOIC-8.1 | 59.37,13.95 59.37,13.02 | 59.37,13.02 59.69,13.02 | 59.37,13.02 59.06,13.02
  Bottom 0.406: EMPTY2.1 62.8,15.94 59.37,19.37
  Bottom 1.27: 59.37,18.57 59.37,19.37 J-SOIC-8.1
TINY/VCC  (via drill 0.7)
  Top 0.813: 87.15,10.95 86.68,10.95 | 86.68,10.95 80.33,10.95 ATTINY.8 80.33,13.34 | 80.33,13.34 v78.42,13.34 | 80.33,13.34 80.33,14.45 | 94.93,20.8 89.38,20.8 89.38,20.64 | 94.93,20.8 PINVCC-18.1 | 61.75,11.59 61.75,11.27 65.88,11.27 65.88,11.91 61.75,11.91 61.75,11.59 | v59.37,11.59 61.75,11.59 | 95.57,20.16 89.38,20.16 89.38,20.64 | 89.38,20.64 95.57,20.64 95.57,20.16 | 96.68,20.8 96.68,86.84 97.31,86.84 97.31,20.8 | 97.31,20.8 96.68,20.8 | 95.57,20.16 97.31,20.16 97.31,20.8 | 94.93,20.8 96.68,20.8 | 54.29,8.57 54.29,11.59 | LED-NAP.A 86.68,10.95 | 54.29,16.35 52.07,16.35 52.07,34.77 36.51,34.77 PINVCC-4.1 | PINVCC-10.1 54.29,24.45
  Top 1.016: TINY-ISP.2 92.39,14.13 87.15,14.13 87.15,10.95 | PINVCC-1.1 PINVCC-2.1 PINVCC-3.1 PINVCC-4.1
  Top 1.27: PINVCC-14.1 54.29,16.35 PINVCC-12.1 PINVCC-11.1 PINVCC-10.1 PINVCC-9.1 | PINVCC-17.1 PINVCC-16.1 PINVCC-15.1 54.29,11.59 PINVCC-14.1 | PINVCC-14.1 PINVCC-13.1 | LED-NAP.A 86.68,10.64
  Top 1.422: 86.68,10.64 86.68,9.84
  Bottom 0.406: PINVCC-17.1 54.29,4.6
  Bottom 0.813: 62.07,11.59 62.07,11.91 65.25,11.91 65.25,11.27 62.07,11.27 | 54.29,4.6 54.29,2.38 46.67,2.38 | 46.67,2.38 PINVCC-7.1 PINVCC-8.1 | 46.67,2.38 26.35,2.38 PINVCC-5.1 PINVCC-6.1
  Bottom 1.27: TINY-ISP.2 94.93,12.38 | 94.93,12.38 C8.1 | v78.42,13.34 78.42,11.59 69.69,11.59 | 69.69,11.59 62.07,11.59 v59.37,11.59 54.29,11.59 | PINVCC-18.1 94.93,12.38 | P-U/PB3.2 P-U/PB4.2 69.69,11.59 | PINVCC-12.1 54.29,16.35 | 54.29,16.35 PINVCC-13.1 54.29,11.59 | 54.29,11.59 PINVCC-16.1 PINVCC-17.1 | 54.29,16.35 54.29,24.45
USB1
  Bottom 1.016: X1.VBUS 13.65,18.59 PINUSB1.1 13.65,15.72 C1.1
USB2
  Bottom 1.016: X1.D- 13.65,21.09 PINUSB2.1
USB3
  Bottom 1.016: X1.D+ 9.53,23.02 11.11,23.02 PINUSB3.1
USB4
  Bottom 1.016: X1.GND 9.53,16.03 11.11,16.03 PINUSB4.1 11.11,15.72 C1.2
(copper drawn outside any net)
  shapes: Bottom circle x4, Top circle x4

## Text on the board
tPlace: F | E | D | C | B | A | 5 | 4 | 4 | 5 | 1 | 2 | 6 | 3 | 3 | 6 | 3 | 7 | 2 | 1 | 1 | 2 | 7 | 4 | F | E | D | C | B | A | 8 | 8 | 9 | 9 | Y | 10 | 10 | X | 5 | 5 | 11 | 11 | W | 12 | 12 | V | 13 | 10 | 10 | 13 | U | 14 | 14 | T | A | B | 15 | 15 | S | 15 | 15 | 16 | 16 | R | 17 | 17 | Q | 18 | 20 | 20 | 18 | P | 19 | 19 | O | 20 | 20 | N | 25 | 25 | 21 | 21 | M | L | 22 | 22 | 23 | 30 | 30 | 23 | K | 24 | 24 | J | 25 | 30 | 31 | 31 | 30 | 25 | I | 26 | 29 | 29 | 28 | 27 | 26 | H | 1.27mm | G | 27 | 28 | HIGH | F | 2mm | E | GND | D | C | Vcc | LOW | B | C | D | A | B3 | B4 | B5 | B2 | B1 | B0 | GND | Vcc | 1 | Vcc | SOIC8 | A | ISP | ATtiny | 1 | GND | Vcc | GND | Vcc | 5 | GND | GND | PB3
bPlace: F | E | D | C | B | A | 5 | 4 | 4 | 5 | ATtiny / protoboard | 17x25 pins / & / SMD PAD | 6 | 3 | 3 | 6 | 7 | 2 | 1 | 1 | 2 | 7 | F | E | D | C | B | A | 8 | 8 | 9 | 9 | Y | 10 | 10 | X | 11 | 11 | W | 12 | 12 | V | 13 | 5 | 5 | 13 | U | 14 | 14 | T | 10 | 10 | A | B | 15 | 15 | S | 16 | 15 | 15 | 16 | R | 17 | 20 | 20 | 17 | Q | 18 | 18 | P | 25 | 25 | 19 | 19 | O | 30 | 30 | 20 | 20 | N | 21 | 0.65mm | 21 | M | L | 22 | 22 | 23 | 23 | K | GND | 24 | 24 | J | 25 | 30 | 31 | 31 | 30 | 25 | I | 26 | 29 | 29 | 26 | H | G | 27 | 28 | 28 | 27 | F | LOW | E | GND | D | C | Vcc | B | B3 | B5 | B2 | B0 | C | D | B4 | B1 | A | 0.5mm | Vcc | TSSOP8 | Vcc | GND | GND | GND | PB3 | Vcc | Vcc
